(* Logix 5000 AddOnInstructionDefinition export NORD_ADC; software revision 24.02; part 3 of 3 *)
(* tags used below, declared in another part *)
   Done : BOOL;
   Busy : BOOL;
   CompletionPercent : DINT;   // Backup/Restore Complete Percentage
   GetID_InProcess : BOOL;
   BackupInProcess : BOOL;
   RestoreInProcess : BOOL;
   GetID_SM : INT;   // 0: Not Active 10: Reset Info 20: Prepare Read Msg 30: Read Trigger 40: Read Complete 41: Store Data 42: Record Error 50:
   BackupSM : INT;   // 0: Not Active 10: Reset indexes 20: Clear Old Backup 30: Reset Indexes 40: Prepare Read Msg 50: Read Trigger 60: Read Co
   RestoreSM : INT;   // 0: Not Active 10: Reset Indexes 15: # of Saved Param 20: Get RestoreParam 21: Prepare Read Msg 22: Read Trigger 23: Read
   AOI_FirstScanONS : BOOL;
(* NORD_ADC, continued *)

ROUTINE Prescan   (* ladder *)
// Prescan
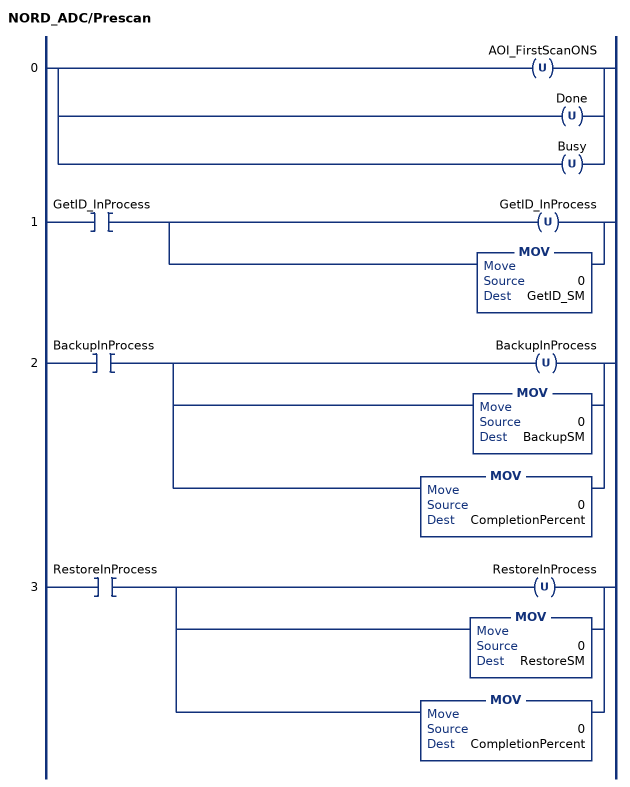
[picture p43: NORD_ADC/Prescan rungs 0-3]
   0: [OTU(AOI_FirstScanONS) ,OTU(Done) ,OTU(Busy) ];
   1: XIC(GetID_InProcess)[OTU(GetID_InProcess) ,MOV(0,GetID_SM) ];
   2: XIC(BackupInProcess)[OTU(BackupInProcess) ,MOV(0,BackupSM) ,MOV(0,CompletionPercent) ];
   3: XIC(RestoreInProcess)[OTU(RestoreInProcess) ,MOV(0,RestoreSM) ,MOV(0,CompletionPercent) ];
END_ROUTINE
END_ADD_ON_INSTRUCTION
